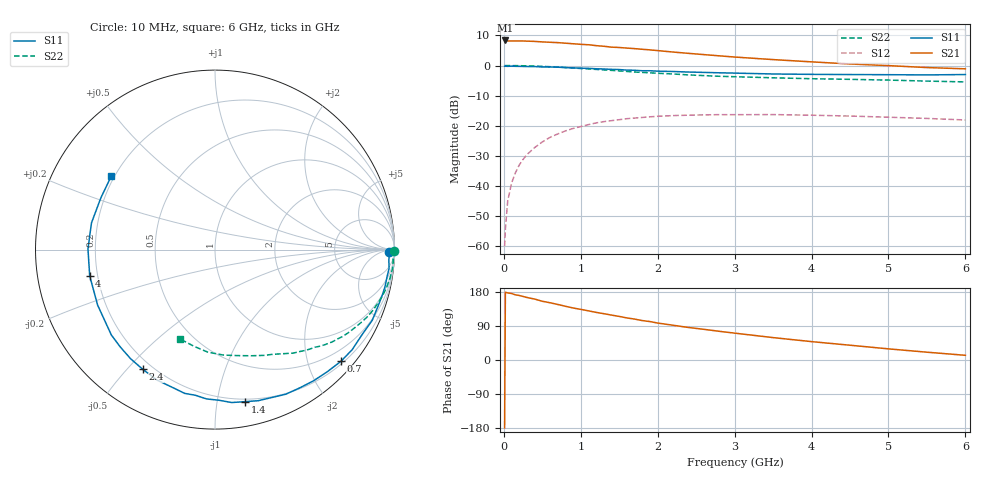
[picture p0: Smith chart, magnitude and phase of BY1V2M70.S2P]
! SIEMENS Small Signal Semiconductors
! BFY420
! Si NPN RF SIEGET Grounded Emitter Transistor in MICRO-X
! VCE = 1.25 V  IC = 0.7 mA
! Common Emitter S-Parameters:  October  1996
# GHz  S  MA  R  50
!  f  S11  S21  S12  S22
! GHz  MAG  ANG  MAG  ANG  MAG  ANG  MAG  ANG
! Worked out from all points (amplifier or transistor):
!   36 points, 10 MHz to 6 GHz, reference 50 ohm
!   highest |S21| = 8.3 dB at 20 MHz (marker M1)
!   |S21| within 3 dB of that: start of sweep to 1.834 GHz
!   unconditionally stable (mu >= 1): 4.69 GHz to end of sweep
!   at 250 MHz: K = 0.03, MSG = 19.7 dB, |S12| = -31.2 dB
!   at 1.4 GHz: K = 0.21, MSG = 12.2 dB, |S12| = -18.3 dB
!   at 6 GHz: K = 1.37, MAG = 4.9 dB, |S12| = -18.1 dB
!   S11 on the Smith chart (normalised r, x): 10 MHz: 59, -25; 700 MHz: 0.25, -2.61; 1.4 GHz: 0.18, -1.20; 2.4 GHz: 0.16, -0.55; 4 GHz: 0.17, -0.10; 6 GHz: 0.19, +0.31
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0.01  0.9715 -0.7  2.605 -179.2  0.001 99.1  0.9999 -0.3
0.02  0.9726 -1.5  2.607 178.7  0.0019 94.3  0.9971 -0.6
0.05  0.97 -3.2  2.56 177.0  0.0056 88.5  0.9985 -1.6
0.1  0.9756 -6.2  2.559 175.6  0.0111 87.1  0.994 -3.1
0.15  0.9705 -9.0  2.555 171.9  0.0165 84.4  0.9957 -4.8
0.2  0.9694 -12.3  2.56 170.3  0.0222 82.4  0.9942 -6.3
0.3  0.9624 -18.2  2.54 165.0  0.0332 79.2  0.9877 -9.4
0.4  0.9606 -24.2  2.516 160.8  0.0433 75.1  0.9791 -12.5
0.5  0.9462 -30.3  2.465 155.0  0.0538 70.8  0.9678 -15.5
0.7  0.9379 -41.6  2.399 146.6  0.073 63.6  0.9417 -21.2
0.9  0.9141 -53.1  2.299 137.3  0.0901 56.2  0.909 -26.6
1.1  0.8971 -63.9  2.212 129.7  0.1044 49.6  0.8769 -31.7
1.4  0.8635 -78.9  2.019 118.5  0.1215 40.5  0.8306 -38.3
1.8  0.8188 -97.7  1.86 104.0  0.1372 30.1  0.7684 -45.9
2.2  0.7955 -113.9  1.674 91.7  0.1474 21.0  0.723 -52.9
2.4  0.779 -121.1  1.592 85.8  0.1497 17.4  0.6981 -56.1
2.8  0.7567 -134.3  1.448 75.7  0.1528 10.4  0.6625 -61.9
3.5  0.7234 -154.7  1.254 59.1  0.1532 1.2  0.6252 -71.1
4  0.7133 -168.2  1.15 48.5  0.1495 -4.5  0.6033 -78.2
4.5  0.7078 179.6  1.06 39.0  0.1448 -9.2  0.5894 -85.5
5.5  0.6982 155.7  0.925 20.6  0.1322 -14.8  0.5512 -102.3
6  0.7082 144.7  0.881 12.4  0.1246 -15.3  0.5341 -111.7
